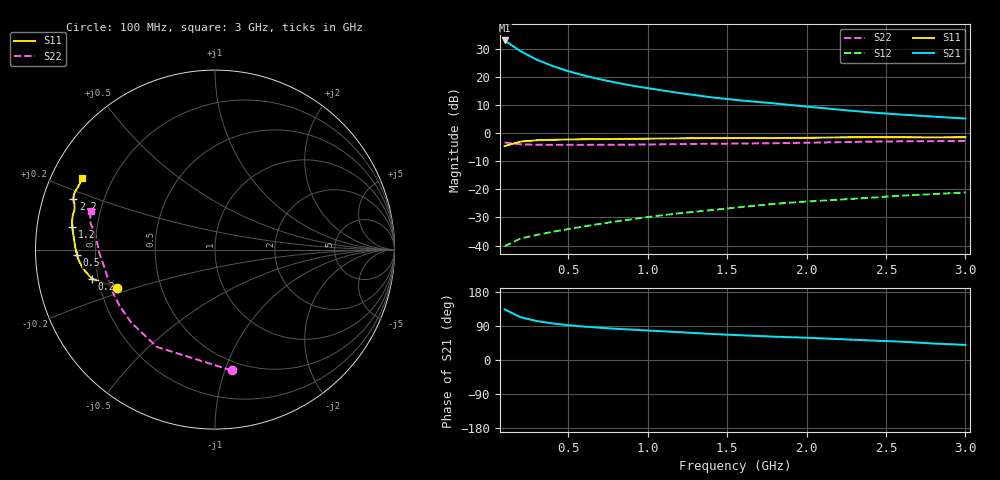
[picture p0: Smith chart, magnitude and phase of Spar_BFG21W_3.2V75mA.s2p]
! Filename: 3_275bfg21.001
! Title: BFG21W
! Bias: Vce=3.2V; Ic=75mA
! Company: NXP Semiconductors NL
! User: Quality&Reliability T&D
! Measure time: 10 Nov 1999 / 11:42:39
#  MHz  S  MA  R 50
! Freq  S11  S21  S12  S22  :
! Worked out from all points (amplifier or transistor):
!   20 points, 100 MHz to 3 GHz, reference 50 ohm
!   highest |S21| = 32.9 dB at 100 MHz (marker M1)
!   |S21| within 3 dB of that: start of sweep to 178.7 MHz
!   unconditionally stable (mu >= 1): 764.4 MHz to end of sweep
!   at 400 MHz: K = 0.80, MSG = 29.5 dB, |S12| = -35.1 dB
!   at 1.2 GHz: K = 1.06, MAG = 19.9 dB, |S12| = -28.5 dB
!   at 3 GHz: K = 1.05, MAG = 11.7 dB, |S12| = -21.1 dB
!   S11 on the Smith chart (normalised r, x): 100 MHz: 0.27, -0.18; 200 MHz: 0.17, -0.11; 500 MHz: 0.13, -0.02; 1.2 GHz: 0.11, +0.08; 2.2 GHz: 0.09, +0.17; 3 GHz: 0.09, +0.25
100  0.586 -158.4  44.29 133.5  0.009755 53.3  0.6794 -82.2
200  0.7058 -166.8  28.55 113.0  0.01331 47.3  0.6317 -120.8
300  0.7433 -171.9  20.3 103.0  0.01544 48.6  0.6191 -139.1
400  0.7596 -175.2  15.6 96.6  0.01751 52.0  0.617 -149.4
500  0.7696 -177.7  12.62 91.9  0.01964 54.9  0.6169 -156.0
600  0.7756 -179.8  10.54 88.2  0.02189 57.8  0.6175 -160.7
700  0.7805 178.4  9.053 85.1  0.02425 60.4  0.6181 -164.3
800  0.7847 176.7  7.898 82.4  0.02681 62.5  0.6195 -167.2
900  0.7896 175.1  7 80.2  0.02935 64.6  0.6225 -169.8
1000  0.795 173.6  6.283 77.9  0.0322 65.9  0.6265 -172.1
1200  0.8053 170.9  5.152 73.4  0.03748 67.7  0.6366 -175.8
1400  0.8119 168.8  4.323 68.7  0.04272 68.8  0.6461 -178.8
1600  0.8153 166.5  3.769 65.0  0.04869 69.7  0.6518 178.6
1800  0.8137 164.1  3.366 61.5  0.05534 70.2  0.6602 175.8
2000  0.8225 162.2  2.958 58.7  0.06058 71.0  0.6723 173.0
2200  0.8387 160.2  2.618 55.2  0.0655 71.1  0.6876 170.6
2400  0.8443 158.4  2.332 51.6  0.07066 70.5  0.7032 168.8
2600  0.8416 156.6  2.13 48.4  0.07736 69.6  0.7134 167.2
2800  0.8375 154.2  1.961 43.4  0.08228 68.1  0.7182 165.1
3000  0.842 151.7  1.812 39.9  0.08815 67.2  0.726 162.6
